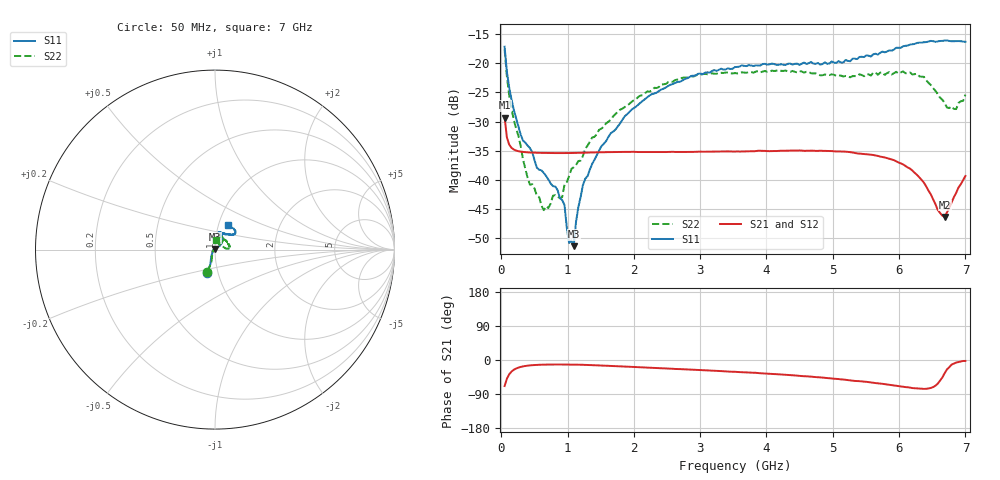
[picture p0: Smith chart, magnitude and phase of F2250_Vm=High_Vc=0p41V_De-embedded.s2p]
! Integrated Device Technology
! Corporate Headquarters
! 6024 Silver Creek Valley Road
! San Jose, CA 95138  USA
! Phone:  1-408-284-8200
! Toll Free:  1-800-223-1366
! Webpage:  http://www.idt.com/
! Timing and RF Division
! 515 Groton Road, Suite 102
! Westford, MA 01886-6024
! Device:  F2250
! Description: Voltage Variable RF Attenuator
! Frequency:  50.0 -  6000.00 MHz
! Package:  3x3 mm Thin QFN Plastic Package: 16 pin
! Ports:  2 RF, 3 DC
!  Pin  1  = GND
!  Pin  2  = NC
!  Pin  3  = RF1  = Port 1
!  Pin  4  = NC
!  Pin  5  = GND
!  Pin  6  = GND
!  Pin  7  = GND
!  Pin  8  = GND
!  Pin  9  = NC
!  Pin 10  = RF2  = Port 2
!  Pin 11  = NC
!  Pin 12  = GND
!  Pin 13  = GND
!  Pin 14  = VCNTRL
!  Pin 15  = VDD
!  Pin 16  = VMODE
! Vcntrl:  0.410 Volts
! Vmode:  +3.300 Volts
! Vdd:  +3.30  Volts
! Current:  1.263 mA
! Data:  The device was measured on a the F2250 evaluation board which has
!  individual transmission lines to the RF pins.  Data was collected
!  using a calibrated network analyzer.  The evaluation board was
!  de-embedded using a TRL calibration technique.
!  The reference plane is the edge of the package pin.
! Misc:  SN 10
!  Action Tracker AT0258
! Date Measured:  2014-11-26
! Date:  2015-10-15  MJV
! Note:
!  Integrated Device Technology supplies this data as a sample of measured
!  data at the package pin for this product.  Your particular data for this
!  product may vary.
!  Data was taken at 25 degrees C.
!  Integrated Device Technology reserves the right to change this data at anytime.
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# GHz S dB R 50
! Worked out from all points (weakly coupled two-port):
!   201 points, 50 MHz to 7 GHz, reference 50 ohm
!   highest |S21| = -29.31 dB at 50 MHz (marker M1); lowest = -46.3 dB at 6.687 GHz (marker M2)
!   lowest |S11| = -51.3 dB at 1.093 GHz (marker M3), VSWR 1.01, Z = 50 + j0.271 ohm
!   |S11| at or under -10 dB: start of sweep to end of sweep
!   |S22| runs from -45.2 to -17.7 dB; largest |S21 - S12| = 4.9e-05
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0.05  -17.17 -108.5  -29.31 -68.7  -29.31 -68.6  -17.65 -109.2
0.1195  -24.20 -111.9  -33.94 -37.7  -33.95 -37.7  -25.55 -109.3
0.29325  -32.27 -127.3  -35.15 -18.2  -35.15 -18.2  -34.22 -120.5
0.43225  -34.54 -145.3  -35.30 -14.2  -35.29 -14.2  -40.82 -156.6
0.5365  -37.90 -154.6  -35.34 -12.9  -35.34 -12.9  -42.70 -174.6
0.64075  -38.80 -162.5  -35.37 -12.2  -35.37 -12.2  -45.17 148.9
0.77975  -41.06 176.3  -35.39 -11.9  -35.39 -11.9  -42.69 119.5
0.91875  -43.45 156.3  -35.39 -11.9  -35.39 -11.9  -42.92 96.8
0.9535  -44.29 170.9  -35.39 -11.9  -35.39 -11.9  -40.79 98.6
1.023  -50.80 140.0  -35.38 -12.0  -35.38 -12.0  -39.33 80.7
1.0925  -51.34 90.0  -35.37 -12.2  -35.37 -12.2  -37.81 73.6
1.12725  -47.16 61.2  -35.36 -12.3  -35.36 -12.3  -37.44 66.6
1.2315  -40.86 40.7  -35.32 -12.7  -35.32 -12.7  -35.87 55.3
1.6485  -32.02 41.1  -35.24 -15.4  -35.24 -15.5  -29.72 49.3
2.37825  -24.75 46.6  -35.20 -21.4  -35.21 -21.4  -24.08 48.4
3.525  -20.65 71.7  -35.14 -31.1  -35.14 -31.2  -21.69 70.1
4.7065  -20.06 72.0  -34.99 -44.5  -34.98 -44.5  -21.76 68.7
5.85325  -17.79 40.5  -36.39 -65.4  -36.39 -65.5  -21.52 20.7
6.3745  -16.40 40.9  -40.46 -76.2  -40.48 -76.2  -22.33 4.4
6.68725  -16.11 47.8  -46.34 -34.7  -46.30 -34.3  -26.79 26.2
6.861  -16.22 54.5  -42.21 -6.8  -42.18 -6.8  -27.86 58.1
7  -16.32 62.4  -39.32 -2.5  -39.29 -2.7  -25.38 86.0
